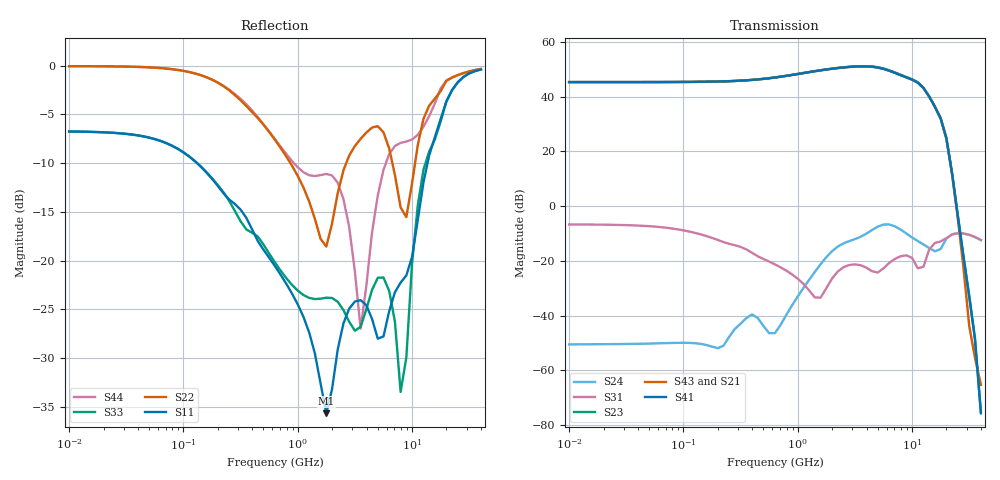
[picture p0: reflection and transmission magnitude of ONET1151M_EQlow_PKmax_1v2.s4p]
! Touchstone Ver. 1.0
! Thu Sep  6 16:04:18 2012
! Number of ports is 4
# Hz	S	DB	R	50.000000
! SCATTERING PARAMETERS  :
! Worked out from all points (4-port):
!   73 points, 10 MHz to 40 GHz, reference 50 ohm
!   strongest paths, dB at 10 MHz, 79.43 MHz, 631 MHz, 5.012 GHz, 40 GHz:
!     S41: 45.3, 45.3, 47.0, 50.6, -75.6
!     S43: 45.3, 45.3, 47.0, 50.6, -65.2
!     S21: 45.3, 45.3, 47.0, 50.8, -65.1
!     S23: 45.3, 45.3, 47.0, 50.7, -75.1
!     S31: -6.7, -8.1, -21.2, -24.2, -12.4
!     S24: -50.5, -49.9, -46.4, -7.5, -12.4
!   lowest |S11| = -35.7 dB at 1.778 GHz (marker M1), VSWR 1.03, Z = 51.1 - j1.25 ohm
!   |S11| at or under -10 dB: 132 MHz to 13.68 GHz (13.55 GHz wide, 196 % of centre)
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1e7  -6.75 -4.6  -110.77 178.1  -6.68 -4.3  -110.74 178.1
     45.32 -175.5  -0.05 7.1  45.32 4.5  -50.48 9.5
     -6.67 -4.3  -110.76 178.1  -6.75 -4.6  -110.76 178.1
     45.31 4.5  -50.37 9.5  45.31 -175.5  -0.05 7.1
1.778279e9  -35.67 -47.9  -39.38 57.1  -25.80 -50.3  -39.31 57.1
            49.96 121.6  -18.55 -56.6  49.95 -58.4  -18.64 56.4
            -29.96 20.3  -39.35 57.1  -23.80 -77.5  -39.31 57.1
            49.91 -58.8  -21.45 -105.5  49.90 121.2  -11.10 -94.5
3.981072e9  -24.57 -87.6  -38.65 -7.1  -26.21 65.3  -38.59 -6.9
            51.13 14.2  -6.86 -117.2  51.13 -165.8  -10.04 -122.7
            -22.45 -71.9  -38.64 -6.7  -24.99 91.1  -38.60 -7.0
            51.05 -166.6  -21.72 53.2  51.04 13.4  -22.58 -80.8
5.623413e9  -27.77 125.1  -37.39 -28.7  -27.47 -2.0  -37.34 -28.4
            50.30 -65.5  -6.84 170.1  50.29 114.5  -6.70 148.5
            -22.70 150.8  -37.36 -28.1  -21.73 -3.3  -37.32 -28.5
            50.14 113.7  -17.49 -142.6  50.13 -66.2  -10.68 -123.5
7.943282e9  -22.25 27.3  -38.12 -63.9  -23.28 97.6  -38.10 -63.5
            48.01 -169.9  -14.54 108.4  47.99 10.2  -8.52 68.1
            -18.28 70.6  -38.12 -63.4  -33.47 -35.4  -38.03 -64.1
            47.85 9.6  -8.08 112.7  47.83 -170.3  -7.91 150.5
1.122018e10  -15.84 24.4  -40.29 -99.9  -18.90 52.0  -40.31 -98.7
             45.26 41.3  -8.14 88.0  45.25 -138.4  -12.71 29.4
             -22.69 32.1  -40.39 -98.3  -14.35 37.7  -40.25 -100.2
             45.12 -139.3  -8.42 19.7  45.09 41.1  -7.10 66.5
4e10  -0.38 -143.6  -68.78 139.4  -12.36 -52.9  -68.59 139.3
      -65.06 -127.0  -0.33 -143.9  -75.06 -54.7  -12.41 -53.2
      -12.36 -52.9  -68.51 138.9  -0.38 -143.5  -68.77 139.6
      -75.64 -62.1  -12.41 -53.3  -65.25 -126.5  -0.33 -143.9
